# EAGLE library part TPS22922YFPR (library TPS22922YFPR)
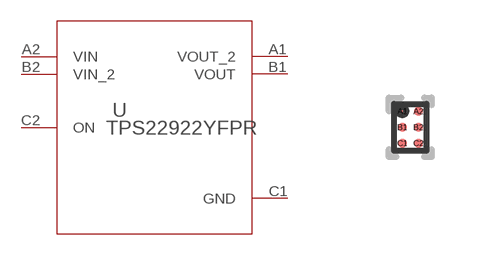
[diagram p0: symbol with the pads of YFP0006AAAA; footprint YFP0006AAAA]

Designator prefix U

## TPS22922YFPR (COMPTYPE: IC; MANUFACTURER: Texas Instruments; MOUNTTYPE: SMT; PACKAGEREFERENCE: YFP0006AAAA; PARTNUMBER: TPS22922YFP; PIN_COUNT: 6; REFDES: RefDes; ROHS: Y; TYPE: TYPE; VALUE: Value)  [YFP0006AAAA]
A1  VOUT_2  out
A2  VIN  in
B1  VOUT  out
B2  VIN_2  in
C1  GND  pwr
C2  ON  in

## Footprint YFP0006AAAA (pad centres in mm)
smd 0.229 x 0.229: A1 -0.2,0.4; A2 0.2,0.4; B1 -0.2,0; B2 0.2,0; C1 -0.2,-0.4; C2 0.2,-0.4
